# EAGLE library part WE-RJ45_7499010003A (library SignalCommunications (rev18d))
WE-RJ45 LAN Transformer Order Code 7499010003A Design THT xBase-T 10/100 Base-T Ports 1x1 Application Standard Tab Position UP LED (Left-Right) NO EMI Fingers No Details see: http://katalog.we-online.de/en/pbs/WE-LAN-RJ45 Created by Yingchun Shan 2016 (C) Wurth Elektronik
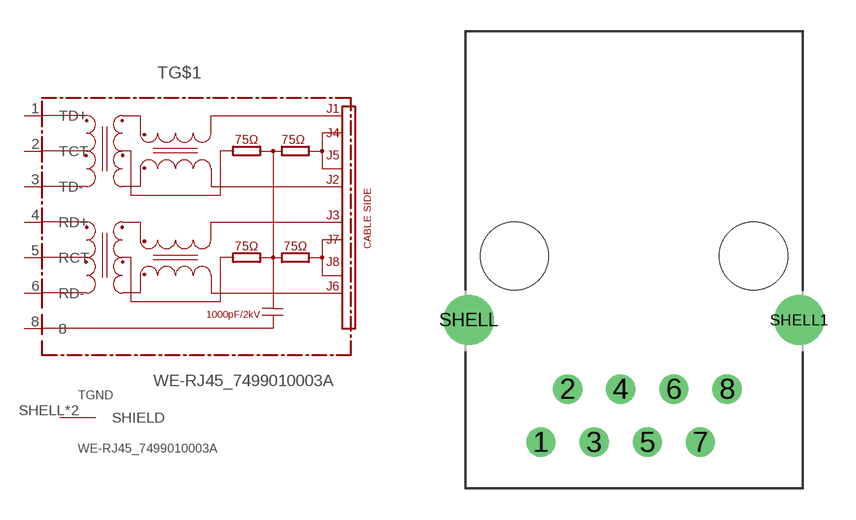
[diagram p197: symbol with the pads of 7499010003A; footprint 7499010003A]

Designator prefix T; gates G$1=7499010003A GND=SHIELD

## WE-RJ45_7499010003A  [7499010003A]
1  G$1:TD+
2  G$1:TCT
3  G$1:TD-
4  G$1:RD+
5  G$1:RCT
6  G$1:RD-
8  G$1:8
SHELL  GND:SHIELD  pas
SHELL1  GND:SHIELD  pas

## Footprint 7499010003A (pad centres in mm)
drill 0.89: 1 -4.445,-5.84; 2 -3.175,-3.3; 3 -1.905,-5.84; 4 -0.635,-3.3; 5 0.635,-5.84; 6 1.905,-3.3; 7 3.175,-5.84; 8 4.445,-3.3
drill 1.6: SHELL -7.9,0; SHELL1 7.9,0
hole 3.25 at -5.715,3.05
hole 3.25 at 5.715,3.05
